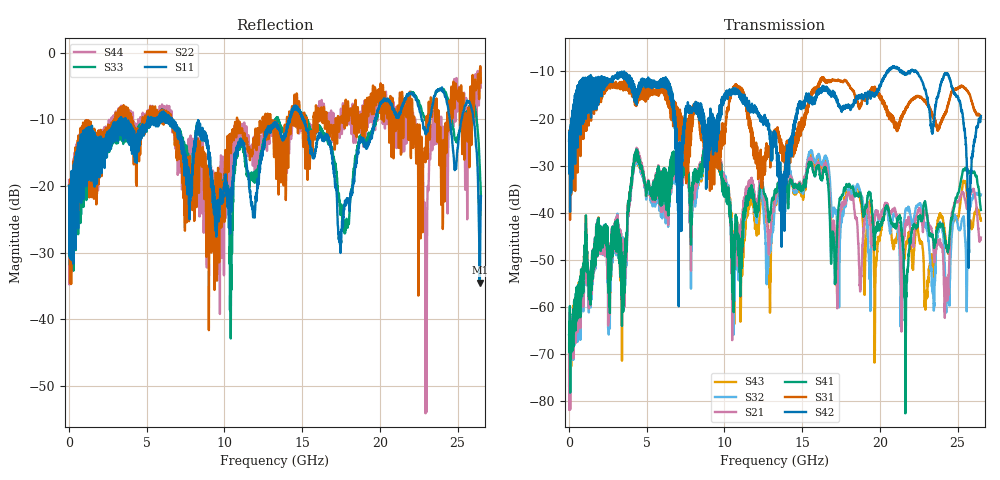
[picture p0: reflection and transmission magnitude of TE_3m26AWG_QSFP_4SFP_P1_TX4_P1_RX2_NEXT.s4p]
!Agilent Technologies,N5222A,MY51421691,A.10.00.00
!Agilent N5222A: A.10.00.00
!Date: Friday, January 30, 2015 12:34:22
!Correction: S11(Full 4 Port(1,2,3,4))
!S12(Full 4 Port(1,2,3,4))
!S13(Full 4 Port(1,2,3,4))
!S14(Full 4 Port(1,2,3,4))
!S21(Full 4 Port(1,2,3,4))
!S22(Full 4 Port(1,2,3,4))
!S23(Full 4 Port(1,2,3,4))
!S24(Full 4 Port(1,2,3,4))
!S31(Full 4 Port(1,2,3,4))
!S32(Full 4 Port(1,2,3,4))
!S33(Full 4 Port(1,2,3,4))
!S34(Full 4 Port(1,2,3,4))
!S41(Full 4 Port(1,2,3,4))
!S42(Full 4 Port(1,2,3,4))
!S43(Full 4 Port(1,2,3,4))
!S44(Full 4 Port(1,2,3,4))
!S4P File: Measurements: <S11,S12,S13,S14>,
!<S21,S22,S23,S24>,
!<S31,S32,S33,S34>,
!<S41,S42,S43,S44>:
# Hz S  dB  R 50.0
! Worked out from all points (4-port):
!   2650 points, 10 MHz to 26.5 GHz, reference 50 ohm
!   strongest paths, dB at 10 MHz, 6.63 GHz, 13.26 GHz, 19.88 GHz, 26.5 GHz:
!     S42: -24.7, -16.1, -25.1, -13.9, -19.5
!     S31: -24.7, -19.1, -23.3, -14.9, -19.7
!     S41: -66.1, -27.7, -35.2, -43.0, -39.4
!     S21: -67.8, -28.1, -36.7, -40.4, -45.3
!     S32: -76.8, -28.7, -38.2, -40.7, -36.1
!     S43: -73.5, -28.2, -37.7, -46.0, -41.7
!   lowest |S11| = -34.5 dB at 26.43 GHz (marker M1), VSWR 1.04, Z = 51 - j1.6 ohm
!   |S11| at or under -10 dB: start of sweep to 3.24 GHz; 6.606 GHz to 14.16 GHz (7.551 GHz wide, 72.7 % of centre); 15.1 GHz to 19.69 GHz (4.582 GHz wide, 26.3 % of centre)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
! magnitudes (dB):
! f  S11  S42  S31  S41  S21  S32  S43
! 10 MHz  -20.0  -24.7  -24.7  -66.1  -67.8  -76.8  -73.5
! 4.32 GHz  -16.3  -16.3  -16.8  -28.3  -28.1  -28.6  -28.9
! 13.77 GHz  -12.8  -33.7  -28.1  -35.4  -37.7  -37.8  -35.6
! 21.66 GHz  -6.8  -10.6  -17.9  -66.4  -42.5  -39.4  -47.4
! 22.93 GHz  -12.2  -14.0  -16.2  -38.0  -39.8  -42.5  -60.6
! 26.43 GHz  -34.5  -20.5  -19.4  -37.5  -45.7  -36.3  -40.9
! 26.5 GHz  -21.5  -19.5  -19.7  -39.4  -45.3  -36.1  -41.7
